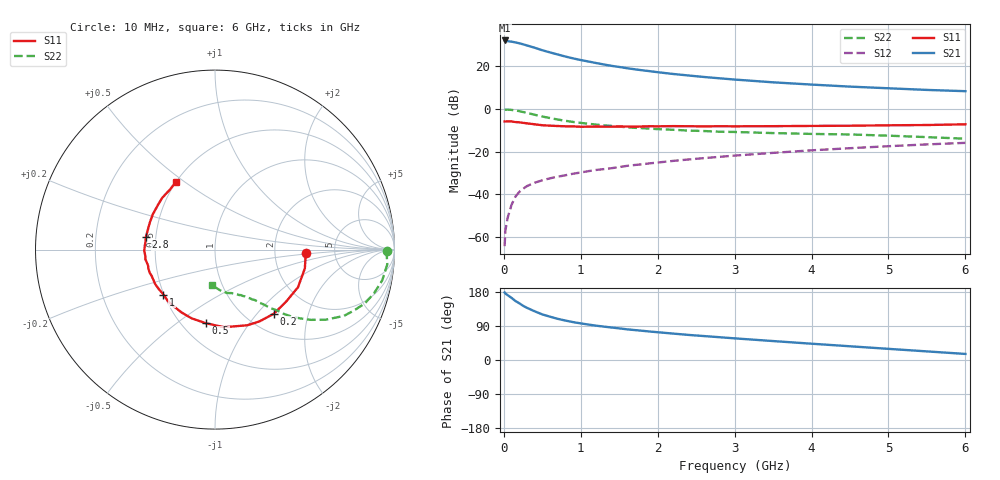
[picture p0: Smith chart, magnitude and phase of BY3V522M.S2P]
! SIEMENS Small Signal Semiconductors
! BFY420
! Si NPN RF SIEGET Grounded Emitter Transistor in MICRO-X
! VCE = 3.5 V  IC = 22 mA
! Common Emitter S-Parameters:  October  1996
# GHz  S  MA  R  50
!  f  S11  S21  S12  S22
! GHz  MAG  ANG  MAG  ANG  MAG  ANG  MAG  ANG
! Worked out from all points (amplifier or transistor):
!   36 points, 10 MHz to 6 GHz, reference 50 ohm
!   highest |S21| = 32.1 dB at 10 MHz (marker M1)
!   |S21| within 3 dB of that: start of sweep to 361.7 MHz
!   unconditionally stable (mu >= 1): start of sweep to 13.98 MHz; 1.953 GHz to end of sweep
!   at 250 MHz: K = 0.31, MSG = 33.9 dB, |S12| = -37.5 dB
!   at 1.4 GHz: K = 0.92, MSG = 24.0 dB, |S12| = -27.8 dB
!   at 6 GHz: K = 1.06, MAG = 10.6 dB, |S12| = -15.9 dB
!   S11 on the Smith chart (normalised r, x): 10 MHz: 3.06, -0.16; 200 MHz: 1.32, -1.23; 500 MHz: 0.65, -0.64; 1 GHz: 0.50, -0.29; 2.8 GHz: 0.44, +0.07; 6 GHz: 0.50, +0.46
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0.01  0.5089 -2.2  40.41 178.2  0.0006 70.2  0.9593 -0.3
0.02  0.5062 -4.7  39.88 175.4  0.0014 70.3  0.9569 -1.5
0.1  0.5078 -24.4  37.92 164.0  0.0056 78.1  0.9471 -10.5
0.15  0.4908 -36.4  36.29 155.8  0.0087 72.7  0.9185 -15.4
0.2  0.485 -47.4  34.74 149.8  0.0112 72.8  0.8867 -19.8
0.25  0.4705 -58.3  32.82 143.1  0.0133 68.7  0.844 -23.8
0.3  0.4582 -67.0  30.89 137.7  0.0154 67.1  0.8077 -27.2
0.4  0.435 -83.4  27.27 128.6  0.0185 62.7  0.7294 -32.4
0.5  0.4134 -97.2  23.81 120.3  0.0211 61.1  0.6627 -36.2
0.6  0.4044 -108.9  21.18 114.3  0.0235 59.7  0.6089 -39.0
0.7  0.3965 -118.3  18.94 108.6  0.0256 60.4  0.5638 -41.3
0.8  0.3904 -126.5  16.94 104.1  0.0277 58.7  0.5257 -43.0
1  0.381 -138.9  14.03 96.6  0.0322 59.6  0.4701 -45.2
1.1  0.3826 -144.8  12.95 93.5  0.0346 59.9  0.4474 -46.6
1.4  0.3821 -157.6  10.24 85.7  0.0406 60.2  0.3985 -49.1
1.6  0.3861 -163.9  9.022 81.0  0.046 59.8  0.3709 -50.9
2.2  0.3943 -179.0  6.607 69.7  0.0602 58.5  0.3237 -55.8
2.8  0.3917 169.7  5.231 60.2  0.0748 55.6  0.2913 -60.4
3.5  0.3931 157.7  4.205 50.0  0.0929 51.4  0.2707 -65.7
4.5  0.4029 142.6  3.334 36.2  0.1196 43.7  0.2513 -74.2
5.5  0.4184 126.7  2.789 22.7  0.1468 34.9  0.2175 -86.6
6  0.4353 119.9  2.605 16.0  0.1596 30.2  0.1997 -94.7
